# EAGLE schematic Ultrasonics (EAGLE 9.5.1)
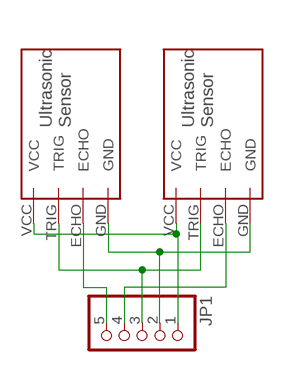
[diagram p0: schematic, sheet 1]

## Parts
JP1  PINHD-1X5  [1X05]
U$1  SEN-15569  [HC-SR04]
U$2  SEN-15569  [HC-SR04]

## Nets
ECHO_L: JP1.5 U$2.ECHO
ECHO_R: JP1.4 U$1.ECHO
GND: JP1.2 U$1.GND U$2.GND
TRIG: JP1.3 U$1.TRIG U$2.TRIG
VDD_5: JP1.1 U$1.VCC U$2.VCC

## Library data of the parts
JP1 = pinhead:PINHD-1X5: PIN HEADER
U$1 U$2 = MILESTONE4LIB_E:SEN-15569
